| Texas Instruments Incorporated
| 6.4-GSPS Single-Channel or 3.2-GSPS Dual-Channel
| 12-Bit RF-Sampling Analog-to-Digital Converter (ADC)
| Marketing part#   ADC12DJ2700AAV, ADC12DJ3200AAV, ADC08DJ3200AAV
| Voltage Range   1.05V - 1.15V & 1.8V - 2.0V
| Package-type   BGA
| #pins/pkg drawing   144-pin AAV
[IBIS Ver]   4.1
[File name]   adc12djxx00aav.ibs
[File Rev]   2.2
[Date]   12/15/2021
| Complete grounds-up generation of the IBIS model, therefore previous revision history deleted.
[Source]   Model built from spectre simulations at:
   Texas Instruments Incorporated.
   12500 TI Blvd
   Dallas, TX -75243
   Support: https://e2e.ti.com/support/data-converters/f/data-converters-forum
[Notes]
   Rev 2.0: 04/15/2021
   - all model data was revised
   - INPUT model now referring to VDD18
   - C_comp data was revised. Currently min and max values are sorted in numerical order
   (otherwise a warning is triggered by the syntax check).
   However, the max. C_comp value is derived for the IBIS min. case
   (high temp., low supply and weak process which leads to max. numerical C_comp value).
   Vice versa for min. C_comp.
   - prior NC models were replaced by TERMINATOR models which cover the clamping behaviour
   - RLC package data was revised
   - Vinl & Vinh in model SYNCB, DEVCLK and SYSREF refer to 1.1V supply
   Rev 2.1: 09/30/2021
   - corrected input pin list
   Rev 2.2: 12/15/2021
   - updates on PECL, LVDS models
   - update on OUTPUT model
[Disclaimer]  This model is designed as an aid for customers of Texas Instruments
 TI and its licensors and suppliers make no warranties, either expressed
 or implied, with respect to this  model, including the warranties of
 merchantability or fitness for a particular purpose.
 The model is provided solely on an "as is" basis. The entire risk as to
 its quality and performance is with the customer.
[Copyright] (C)Copyright 2021 Texas Instruments Incorporated.
   All rights reserved.
[Component]   ADC12DJxx00AAV_PECL   | PECL input on SYNCB, DEVCLK, SYSREF
[Manufacturer]  Texas Instruments Incorporated
[Package]   |144-pin BGA AAV package
|   typ   min   max
R_pkg   0.176   0.01   0.4408
L_pkg   1.97n   0.64n   3.46n
C_pkg   0.63p   0.20p   1.31p
[Pin]   signal_name   model_name   R_pin   L_pin   C_pin
A1   AGND   GND
A2   AGND   GND
A3   AGND   GND
A4   INA+   ADCINCLAMP   0.28155  2.707E-09  6.986E-13
A5   INA-   ADCINCLAMP   0.28375  2.697E-09  6.967E-13
A6   AGND   GND
A7   AGND   GND
A8   DA3+   DXCLAMP   0.21236  2.387E-09  6.418E-13
A9   DA3-   DXCLAMP   0.23082  2.406E-09  6.764E-13
A10   DA2+   DXCLAMP   0.27772  2.658E-09  7.482E-13
A11   DA2-   DXCLAMP   0.30299  2.763E-09  7.886E-13
A12   DGND   GND
B1   TMSTP+   SYNCB_PECL   0.36537  3.376E-09  1.069E-12
B2   AGND   GND
B3   AGND   GND
B4   AGND   GND
B5   AGND   GND
B6   AGND   GND
B7   AGND   GND
B8   DA7+   DXCLAMP   0.15104  1.789E-09  5.369E-13
B9   DA7-   DXCLAMP   0.16987  1.841E-09  5.682E-13
B10   DA6+   DXCLAMP   0.17353  1.861E-09  5.746E-13
B11   DA6-   DXCLAMP   0.19518  2.001E-09  6.161E-13
B12   DGND   GND
C1   TMSTP-   SYNCB_PECL   0.35697  3.459E-09  9.983E-13
C2   SYNCSE\   INPUT   0.18798  2.727E-09  8.975E-13
C3   BG   BGCLAMP   0.05533  9.587E-10  4.058E-13
C4   VA19   POWER
C5   VA11   POWER
C6   AGND   GND
C7   NCOA0   INPUT   0.06384  1.151E-09  4.756E-13
C8   ORA0   OUTPUT   0.05753  1.211E-09  2.050E-13
C9   VD11   POWER
C10   VD11   POWER
C11   DA5+   DXCLAMP   0.16309  1.778E-09  5.434E-13
C12   DA1+   DXCLAMP   0.20396  2.069E-09  6.086E-13
D1   AGND   GND
D2   VA11   POWER
D3   VA11   POWER
D4   VA19   POWER
D5   VA11   POWER
D6   AGND   GND
D7   NCOA1   INPUT   0.01599  7.110E-10  4.255E-13
D8   ORA1   OUTPUT   0.01018  6.389E-10  2.871E-13
D9   DGND   GND
D10   DGND   GND
D11   DA5-   DXCLAMP   0.17735  1.895E-09  5.721E-13
D12   DA1-   DXCLAMP   0.21853  2.226E-09  6.444E-13
E1   AGND   GND
E2   VA19   POWER
E3   VA19   POWER
E4   VA19   POWER
E5   VA11   POWER
E6   AGND   GND
E7   CALTRIG   INPUT   0.06787  1.302E-09  6.170E-13
E8   SCS\   INPUT   0.0709   2.113E-09  6.270E-13
E9   VD11   POWER
E10   VD11   POWER
E11   DA4+   DXCLAMP   0.11035  1.378E-09  4.552E-13
E12   DA0+   DXCLAMP   0.17471  1.835E-09  5.964E-13
F1   CLK+   DEVCLK_PECL   0.44071  3.463E-09  1.223E-12
F2   AGND   GND
F3   AGND   GND
F4   VA19   POWER
F5   VA11   POWER
F6   AGND   GND
F7   CALSTAT   OUTPUT   0.06324  1.881E-09  4.773E-13
F8   SCLK   INPUT   0.05323  1.776E-09  4.600E-13
F9   DGND   GND
F10   DGND   GND
F11   DA4-   DXCLAMP   0.12255  1.392E-09  4.955E-13
F12   DA0-   DXCLAMP   0.18679  1.921E-09  6.051E-13
G1   CLK-   DEVCLK_PECL   0.437   3.145E-09  1.312E-12
G2   AGND   GND
G3   AGND   GND
G4   VA19   POWER
G5   VA11   POWER
G6   AGND   GND
G7   VD11   POWER
G8   SDI   INPUT   0.05979  1.759E-09  5.013E-13
G9   DGND   GND
G10   DGND   GND
G11   DB4-   DXCLAMP   0.12025  1.381E-09  4.906E-13
G12   DB0-   DXCLAMP   0.18571  1.903E-09  5.986E-13
H1   AGND   GND
H2   VA19   POWER
H3   VA19   POWER
H4   VA19   POWER
H5   VA11   POWER
H6   AGND   GND
H7   VD11   POWER
H8   SDO   OUTPUT   0.04215  1.257E-09  3.757E-13
H9   VD11   POWER
H10   VD11   POWER
H11   DB4+   DXCLAMP   0.10716  1.397E-09  4.466E-13
H12   DB0+   DXCLAMP   0.17179  1.810E-09  5.866E-13
J1   AGND   GND
J2   VA11   POWER
J3   VA11   POWER
J4   VA19   POWER
J5   VA11   POWER
J6   AGND   GND
J7   NCOB1   INPUT   0.02676  8.066E-10  4.564E-13
J8   ORB1   OUTPUT   0.03694  9.371E-10  2.044E-13
J9   DGND   GND
J10   DGND   GND
J11   DB5-   DXCLAMP   0.17534  1.869E-09  5.672E-13
J12   DB1-   DXCLAMP   0.21589  2.204E-09  6.396E-13
K1   SYSREF+   SYSREF_PECL   0.35639  2.727E-09  1.127E-12
K2   TDIODE+   TDCLAMP   0.09252  1.752E-09  9.795E-13
K3   TDIODE-   TDCLAMP   0.08963  1.633E-09  9.228E-13
K4   VA19   POWER
K5   VA11   POWER
K6   PD   INPUT   0.14212  2.291E-09  5.856E-13
K7   NCOB0   INPUT   0.07097  1.118E-09  4.550E-13
K8   ORB0   OUTPUT   0.06984  1.405E-09  2.178E-13
K9   VD11   POWER
K10   VD11   POWER
K11   DB5+   DXCLAMP   0.16566  1.794E-09  5.462E-13
K12   DB1+   DXCLAMP   0.20215  2.091E-09  6.106E-13
L1   SYSREF-   SYSREF_PECL   0.36691  2.720E-09  1.103E-12
L2   AGND   GND
L3   AGND   GND
L4   AGND   GND
L5   AGND   GND
L6   AGND   GND
L7   AGND   GND
L8   DB7+   DXCLAMP   0.13435  1.680E-09  5.095E-13
L9   DB7-   DXCLAMP   0.15554  1.732E-09  5.454E-13
L10   DB6+   DXCLAMP   0.17686  1.856E-09  5.789E-13
L11   DB6-   DXCLAMP   0.19951  1.991E-09  6.230E-13
L12   DGND   GND
M1   AGND   GND
M2   AGND   GND
M3   AGND   GND
M4   INB+   ADCINCLAMP   0.2817   2.554E-09  7.079E-13
M5   INB-   ADCINCLAMP   0.28398  2.579E-09  7.223E-13
M6   AGND   GND
M7   AGND   GND
M8   DB3+   DXCLAMP   0.20854  2.351E-09  6.389E-13
M9   DB3-   DXCLAMP   0.2316   2.393E-09  6.824E-13
M10   DB2+   DXCLAMP   0.27749  2.624E-09  7.525E-13
M11   DB2-   DXCLAMP   0.29995  2.762E-09  7.839E-13
M12   DGND   GND
[Diff pin]  inv_pin  vdiff  tdelay_typ  tdelay_min  tdelay_max
A4   A5   0.0   0.0s   0.0s   0.0s   | INA
A8   A9   0.0   0.0s   0.0s   0.0s   | DA3
A10   A11   0.0   0.0s   0.0s   0.0s   | DA2
B8   B9   0.0   0.0s   0.0s   0.0s   | DA7
B10   B11   0.0   0.0s   0.0s   0.0s   | DA6
B1   C1   0.0   0.0s   0.0s   0.0s   | TMSTP
C11   D11   0.0   0.0s   0.0s   0.0s   | DA5
C12   D12   0.0   0.0s   0.0s   0.0s   | DA1
E11   F11   0.0   0.0s   0.0s   0.0s   | DA4
E12   F12   0.0   0.0s   0.0s   0.0s   | DA0
F1   G1   0.0   0.0s   0.0s   0.0s   | CLK
H11   G11   0.0   0.0s   0.0s   0.0s   | DB4
H12   G12   0.0   0.0s   0.0s   0.0s   | DB0
K11   J11   0.0   0.0s   0.0s   0.0s   | DB5
K12   J12   0.0   0.0s   0.0s   0.0s   | DB1
K1   L1   0.0   0.0s   0.0s   0.0s   | SYSREF
L8   L9   0.0   0.0s   0.0s   0.0s   | DB7
L10   L11   0.0   0.0s   0.0s   0.0s   | DB6
M4   M5   0.0   0.0s   0.0s   0.0s   | INB
M8   M9   0.0   0.0s   0.0s   0.0s   | DB3
M10   M11   0.0   0.0s   0.0s   0.0s   | DB2
[Component]   ADC12DJxx00AAV_LVDS   | 100 Ohm termination on SYNCB, DEVCLK, SYSREF
[Manufacturer]  Texas Instruments Incorporated
[Package]   |144-pin BGA AAV package
|   typ   min   max
R_pkg   0.176   0.01   0.4408
L_pkg   1.97n   0.64n   3.46n
C_pkg   0.63p   0.20p   1.31p
[Pin]   signal_name   model_name   R_pin   L_pin   C_pin
A1   AGND   GND
A2   AGND   GND
A3   AGND   GND
A4   INA+   ADCINCLAMP   0.28155  2.707E-09  6.986E-13
A5   INA-   ADCINCLAMP   0.28375  2.697E-09  6.967E-13
A6   AGND   GND
A7   AGND   GND
A8   DA3+   DXCLAMP   0.21236  2.387E-09  6.418E-13
A9   DA3-   DXCLAMP   0.23082  2.406E-09  6.764E-13
A10   DA2+   DXCLAMP   0.27772  2.658E-09  7.482E-13
A11   DA2-   DXCLAMP   0.30299  2.763E-09  7.886E-13
A12   DGND   GND
B1   TMSTP+   SYNCB_LVDS   0.36537  3.376E-09  1.069E-12
B2   AGND   GND
B3   AGND   GND
B4   AGND   GND
B5   AGND   GND
B6   AGND   GND
B7   AGND   GND
B8   DA7+   DXCLAMP   0.15104  1.789E-09  5.369E-13
B9   DA7-   DXCLAMP   0.16987  1.841E-09  5.682E-13
B10   DA6+   DXCLAMP   0.17353  1.861E-09  5.746E-13
B11   DA6-   DXCLAMP   0.19518  2.001E-09  6.161E-13
B12   DGND   GND
C1   TMSTP-   SYNCB_LVDS   0.35697  3.459E-09  9.983E-13
C2   SYNCSE\   INPUT   0.18798  2.727E-09  8.975E-13
C3   BG   BGCLAMP   0.05533  9.587E-10  4.058E-13
C4   VA19   POWER
C5   VA11   POWER
C6   AGND   GND
C7   NCOA0   INPUT   0.06384  1.151E-09  4.756E-13
C8   ORA0   OUTPUT   0.05753  1.211E-09  2.050E-13
C9   VD11   POWER
C10   VD11   POWER
C11   DA5+   DXCLAMP   0.16309  1.778E-09  5.434E-13
C12   DA1+   DXCLAMP   0.20396  2.069E-09  6.086E-13
D1   AGND   GND
D2   VA11   POWER
D3   VA11   POWER
D4   VA19   POWER
D5   VA11   POWER
D6   AGND   GND
D7   NCOA1   INPUT   0.01599  7.110E-10  4.255E-13
D8   ORA1   OUTPUT   0.01018  6.389E-10  2.871E-13
D9   DGND   GND
D10   DGND   GND
D11   DA5-   DXCLAMP   0.17735  1.895E-09  5.721E-13
D12   DA1-   DXCLAMP   0.21853  2.226E-09  6.444E-13
E1   AGND   GND
E2   VA19   POWER
E3   VA19   POWER
E4   VA19   POWER
E5   VA11   POWER
E6   AGND   GND
E7   CALTRIG   INPUT   0.06787  1.302E-09  6.170E-13
E8   SCS\   INPUT   0.0709   2.113E-09  6.270E-13
E9   VD11   POWER
E10   VD11   POWER
E11   DA4+   DXCLAMP   0.11035  1.378E-09  4.552E-13
E12   DA0+   DXCLAMP   0.17471  1.835E-09  5.964E-13
F1   CLK+   DEVCLK_LVDS   0.44071  3.463E-09  1.223E-12
F2   AGND   GND
F3   AGND   GND
F4   VA19   POWER
F5   VA11   POWER
F6   AGND   GND
F7   CALSTAT   OUTPUT   0.06324  1.881E-09  4.773E-13
F8   SCLK   INPUT   0.05323  1.776E-09  4.600E-13
F9   DGND   GND
F10   DGND   GND
F11   DA4-   DXCLAMP   0.12255  1.392E-09  4.955E-13
F12   DA0-   DXCLAMP   0.18679  1.921E-09  6.051E-13
G1   CLK-   DEVCLK_LVDS   0.437   3.145E-09  1.312E-12
G2   AGND   GND
G3   AGND   GND
G4   VA19   POWER
G5   VA11   POWER
G6   AGND   GND
G7   VD11   POWER
G8   SDI   INPUT   0.05979  1.759E-09  5.013E-13
G9   DGND   GND
G10   DGND   GND
G11   DB4-   DXCLAMP   0.12025  1.381E-09  4.906E-13
G12   DB0-   DXCLAMP   0.18571  1.903E-09  5.986E-13
H1   AGND   GND
H2   VA19   POWER
H3   VA19   POWER
H4   VA19   POWER
H5   VA11   POWER
H6   AGND   GND
H7   VD11   POWER
H8   SDO   OUTPUT   0.04215  1.257E-09  3.757E-13
H9   VD11   POWER
H10   VD11   POWER
H11   DB4+   DXCLAMP   0.10716  1.397E-09  4.466E-13
H12   DB0+   DXCLAMP   0.17179  1.810E-09  5.866E-13
J1   AGND   GND
J2   VA11   POWER
J3   VA11   POWER
J4   VA19   POWER
J5   VA11   POWER
J6   AGND   GND
J7   NCOB1   INPUT   0.02676  8.066E-10  4.564E-13
J8   ORB1   OUTPUT   0.03694  9.371E-10  2.044E-13
J9   DGND   GND
J10   DGND   GND
J11   DB5-   DXCLAMP   0.17534  1.869E-09  5.672E-13
J12   DB1-   DXCLAMP   0.21589  2.204E-09  6.396E-13
K1   SYSREF+   SYSREF_LVDS   0.35639  2.727E-09  1.127E-12
K2   TDIODE+   TDCLAMP   0.09252  1.752E-09  9.795E-13
K3   TDIODE-   TDCLAMP   0.08963  1.633E-09  9.228E-13
K4   VA19   POWER
K5   VA11   POWER
K6   PD   INPUT   0.14212  2.291E-09  5.856E-13
K7   NCOB0   INPUT   0.07097  1.118E-09  4.550E-13
K8   ORB0   OUTPUT   0.06984  1.405E-09  2.178E-13
K9   VD11   POWER
K10   VD11   POWER
K11   DB5+   DXCLAMP   0.16566  1.794E-09  5.462E-13
K12   DB1+   DXCLAMP   0.20215  2.091E-09  6.106E-13
L1   SYSREF-   SYSREF_LVDS   0.36691  2.720E-09  1.103E-12
L2   AGND   GND
L3   AGND   GND
L4   AGND   GND
L5   AGND   GND
L6   AGND   GND
L7   AGND   GND
L8   DB7+   DXCLAMP   0.13435  1.680E-09  5.095E-13
L9   DB7-   DXCLAMP   0.15554  1.732E-09  5.454E-13
L10   DB6+   DXCLAMP   0.17686  1.856E-09  5.789E-13
L11   DB6-   DXCLAMP   0.19951  1.991E-09  6.230E-13
L12   DGND   GND
M1   AGND   GND
M2   AGND   GND
M3   AGND   GND
M4   INB+   ADCINCLAMP   0.2817   2.554E-09  7.079E-13
M5   INB-   ADCINCLAMP   0.28398  2.579E-09  7.223E-13
M6   AGND   GND
M7   AGND   GND
M8   DB3+   DXCLAMP   0.20854  2.351E-09  6.389E-13
M9   DB3-   DXCLAMP   0.2316   2.393E-09  6.824E-13
M10   DB2+   DXCLAMP   0.27749  2.624E-09  7.525E-13
M11   DB2-   DXCLAMP   0.29995  2.762E-09  7.839E-13
M12   DGND   GND
[Diff pin]  inv_pin  vdiff  tdelay_typ  tdelay_min  tdelay_max
A4   A5   0.0   0.0s   0.0s   0.0s   | INA
A8   A9   0.0   0.0s   0.0s   0.0s   | DA3
A10   A11   0.0   0.0s   0.0s   0.0s   | DA2
B8   B9   0.0   0.0s   0.0s   0.0s   | DA7
B10   B11   0.0   0.0s   0.0s   0.0s   | DA6
B1   C1   0.0   0.0s   0.0s   0.0s   | TMSTP
C11   D11   0.0   0.0s   0.0s   0.0s   | DA5
C12   D12   0.0   0.0s   0.0s   0.0s   | DA1
E11   F11   0.0   0.0s   0.0s   0.0s   | DA4
E12   F12   0.0   0.0s   0.0s   0.0s   | DA0
F1   G1   0.0   0.0s   0.0s   0.0s   | CLK
H11   G11   0.0   0.0s   0.0s   0.0s   | DB4
H12   G12   0.0   0.0s   0.0s   0.0s   | DB0
K11   J11   0.0   0.0s   0.0s   0.0s   | DB5
K12   J12   0.0   0.0s   0.0s   0.0s   | DB1
K1   L1   0.0   0.0s   0.0s   0.0s   | SYSREF
L8   L9   0.0   0.0s   0.0s   0.0s   | DB7
L10   L11   0.0   0.0s   0.0s   0.0s   | DB6
M4   M5   0.0   0.0s   0.0s   0.0s   | INB
M8   M9   0.0   0.0s   0.0s   0.0s   | DB3
M10   M11   0.0   0.0s   0.0s   0.0s   | DB2
[Series Pin Mapping]   pin_2   model_name   function_table_group
B1   C1   100_Ohm   | SYNCB with 100 Ohm termination
F1   G1   100_Ohm   | DEVCLK with 100 Ohm termination
K1   L1   100_Ohm   | SYSREF with 100 Ohm termination
[Model] 100_Ohm
Model_type Series
Polarity Non-Inverting
Enable Active-High
|   typ   min   max
C_comp   0   0   0
[Voltage Range]   1.10V   1.05V   1.15V
[Temperature Range]  25   125   -40
[R Series]   100   80   120
| Models and submodels in the file (13): SYNCB_LVDS (Input), SYNCB_PECL (Input), DEVCLK_LVDS (Input), DEVCLK_PECL (Input), SYSREF_LVDS (Input), SYSREF_PECL (Input), INPUT (Input), OUTPUT (3-state), DXCLAMP (Terminator), BGCLAMP (Terminator), TDCLAMP (Terminator), ADCINCLAMP (Terminator), 100_Ohm (Series)
